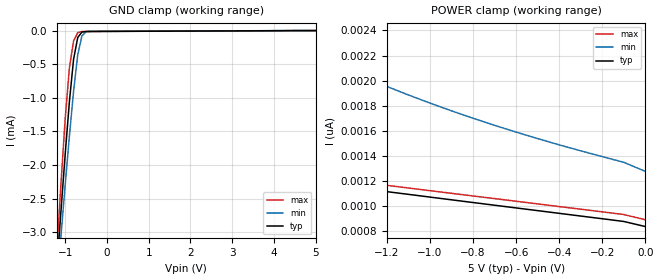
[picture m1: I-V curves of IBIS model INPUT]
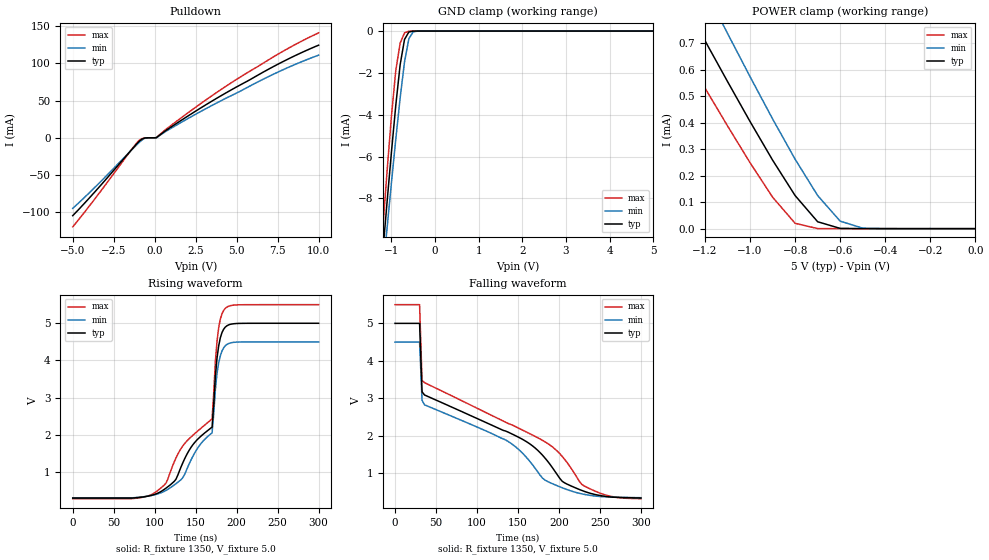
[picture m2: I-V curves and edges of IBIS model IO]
|   PERICOM SEMICONDUCTOR CORP
|   IBIS Model of PI6ULS5V9511A
|   Product Family: ULS
|   MSOP-8 (U) Package
[IBIS Ver] 3.2
[Comment char] |_char
[File Name] pi6uls5v9511a_u_50v.ibs
[File Rev] 1.0
[Source] File originated at Pericom Semiconductor Corp.
[Date] 08/30/2017
[Disclaimer] (C) Copyright PERICOM Semiconductor Corporation
   All rights reserved
  Pericom Semiconductor Corporation hereby grants the user of
  this IBIS model a non-exclusive, nontransferable license to
  use this IBIS model under the following terms.
  This IBIS model is provided on an "AS IS" basis and Pericom
  makes absolutely no warranty with respect to the information
  contained herein. PERICOM DISCLAIMS AND CUSTOMER WAIVES ALL
  WARRANTIES, EXPRESSED OR IMPLIED, INCLUDING WARRANTIES OF
  MERCHANTABILITY OR FITNESS FOR A PARTICULAR PURPOSE. The
  entire risk as to quality and performance is with the customer.
  Accordingly, in no event shall the company be liable for any
  damages, whether in contract or tort, including any lost
  profits or other incidental, consequential, exemplary, or
  punitive damages arising out of the use or application of the
  IBIS model provided in this package. Further, Pericom reserves
  the right to make changes without notice to any product herein
  to improve reliability, function, or design. Pericom does not
  convey any license under patent rights or any other intellectual
  property rights, including those of third parties.
  The user is granted this license only to use the IBIS model
  and is not granted rights to sell, load, rent, lease or license
  the IBIS model in whole or in part, or in modified form to anyone
  other than user. User may modify the IBIS model to suit its specific
  application but rights to derivative works and such modifications
  shall belong to Pericom.
  Pericom is not obligated to provide maintenance or support
  for the licensed IBIS model.
  Contact Pericom at ATTN: APPLICATION ENGINEERING / IBIS MODELS
  1545 Barber Lane Milpitas, CA 95035 USA.
[Component] PI6ULS5V9511A
[Manufacturer] Pericom Semiconductor Corp.
[Package]
| variable   typ   min   max
R_pkg   0.04200   0.03995   0.04405
L_pkg   2.30669n   2.21200n   2.40138n
C_pkg   0.21108p   0.20715p   0.21500p
[Pin] signal_name  model_name   R_pin   L_pin   C_pin
1   ENABLE   INPUT   0.04405   2.40138n   0.21500p
2   SCLOUT   IO   0.03995   2.21200n   0.20715p
3   SCLIN   IO   0.03995   2.21200n   0.20715p
4   GND   GND   0.04405   2.40138n   0.21500p
5   READY   NC   0.04405   2.40138n   0.21500p
6   SDAIN   IO   0.03995   2.21200n   0.20715p
7   SDAOUT   IO   0.03995   2.21200n   0.20715p
8   VCC   POWER   0.04405   2.40138n   0.21500p
| Models and submodels in the file (2): INPUT (Input), IO (Open_drain)
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[Model] INPUT
Model_type Input
Vinl = 1.5000V
Vinh = 3.5000V
| variable   typ   min   max
C_comp   1.600pF   1.560pF   1.640pF
[Voltage Range]   5.0000V   4.5000V   5.5000V
[POWER Clamp Reference] 5.0000V   4.5000V   5.5000V
[GND Clamp Reference]   0.0000V   0.0000V   0.0000V
[Temperature Range]   25   85   -40
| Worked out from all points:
|   GND clamp passes 1 mA (typ) near -0.89 V on its own axis
[GND Clamp]
| Voltage   I(typ)   I(min)   I(max)
-5V       -36.92mA   -32.97mA   -43.67mA
-1.2V     -3.523mA   -3.797mA   -3.27mA
-1.1V     -2.661mA   -3.034mA   -2.251mA
-1V       -1.828mA   -2.287mA   -1.302mA
-900mV    -1.053mA   -1.567mA   -550.5uA
-800mV    -425.6uA   -900.4uA   -153.8uA
-700mV    -102uA     -358.3uA   -30.67uA
-600mV    -22.33uA   -78.81uA   -14.18uA
-500mV    -13.71uA   -18.96uA   -13uA
5V        837.4pA    1.539nA    -201.8pA
[POWER Clamp]
| Voltage   I(typ)   I(min)   I(max)
-5V       2.03nA     9.83nA     1.97nA
-4.4V     1.867nA    7.474nA    1.843nA
-3.5V     1.641nA    4.974nA    1.652nA
-1.8V     1.248nA    2.439nA    1.293nA
-1.7V     1.226nA    2.348nA    1.272nA
-1.4V     1.16nA     2.1nA      1.208nA
-1.2V     1.116nA    1.954nA    1.166nA
-1V       1.073nA    1.821nA    1.124nA
-800mV    1.029nA    1.701nA    1.082nA
-600mV    986.2pA    1.59nA     1.039nA
-100mV    878.2pA    1.349nA    933.7pA
0V        837.7pA    1.277nA    891.7pA
[Model] IO
Model_type Open_drain
Vref=5.000
Rref=1.350E+03
Vmeas=2.50E+00
| variable   typ   min   max
C_comp   4.300E-12   4.290E-12   4.310E-12
[Voltage Range]   5.000E+00   4.500E+00   5.500E+00
[POWER Clamp Reference] 5.000E+00   4.500E+00   5.500E+00
[GND Clamp Reference]   0.000E+00   0.000E+00   0.000E+00
[Pullup Reference]   5.000E+00   4.500E+00   5.500E+00
[Pulldown Reference]   0.000E+00   0.000E+00   0.000E+00
[Temperature Range]   25   85   -40
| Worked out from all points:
|   slope of the pulldown table from 0 to 0.75 V, typ, clamps not added: 69.3 ohm
|   GND clamp passes 1 mA (typ) near -0.75 V on its own axis
|   POWER clamp passes 1 mA (typ) near -1.39 V on its own axis
|   rising waveform, R_fixture 1350, V_fixture 5.0: 20-80 % time 41.9ns typ, 35.5ns min, 50.9ns max; typ from 0.301 V to 5 V
|   falling waveform, R_fixture 1350, V_fixture 5.0: 20-80 % time 156ns typ, 138ns min, 176ns max; typ from 5 V to 0.333 V
[GND Clamp]
| Time   V(typ)   V(min)   V(max)
-5V       -104.6mA   -94.77mA   -119.6mA
-1.2V     -10.63mA   -11.63mA   -9.52mA
-1.1V     -8.183mA   -9.429mA   -6.716mA
-1V       -5.8mA     -7.269mA   -4.08mA
-900mV    -3.55mA    -5.173mA   -1.885mA
-800mV    -1.611mA   -3.196mA   -575.8uA
-700mV    -399.9uA   -1.479mA   -85.6uA
-600mV    -45.37uA   -362.7uA   -5.119uA
-500mV    -3.322uA   -35.76uA   -156.6nA
-400mV    -173.5nA   -2.547uA   -3.218nA
5V        126.9pA    1.739uA    123.8pA
[POWER Clamp]
| Voltage   I(typ)   I(min)   I(max)
-5V       6.861mA    7.517mA    6.252mA
-1.4V     1.023mA    1.241mA    822.9uA
-1.3V     865.9uA    1.071mA    676.4uA
-1.2V     709.9uA    903.6uA    531.2uA
-1.1V     555.7uA    737.5uA    388.2uA
-1V       404.6uA    574uA      249.1uA
-900mV    258.9uA    414.5uA    119uA
-800mV    124.9uA    262.2uA    20.17uA
-700mV    26.02uA    125.1uA    252.6nA
-600mV    923.4nA    28.27uA    1.807nA
-500mV    18.49nA    1.739uA    164.1pA
0V        126.9pA    183.6pA    138.5pA
[Pulldown]
| Voltage   I(typ)   I(min)   I(max)
-5V       -104.6mA   -94.78mA   -119.6mA
-3.5V     -68.93mA   -63.3mA    -77.65mA
-1.4V     -15.73mA   -16.16mA   -15.45mA
-950mV    -4.918mA   -6.353mA   -3.55mA
-800mV    -2.107mA   -3.413mA   -1.333mA
-500mV    -106.5uA   -226.5uA   -70.81uA
100mV     100.4uA    -38.8uA    307.1uA
700mV     10.06mA    8.868mA    11.58mA
2.2V      31.63mA    27.93mA    36.25mA
4.75V     65.28mA    57.45mA    74.97mA
7.6V      99.73mA    89.02mA    113.3mA
10V       124.3mA    111mA      140.9mA
[Rising Waveform]
R_fixture = 1350
V_fixture = 5.0
V_fixture_min = 4.50
V_fixture_max = 5.50
| Time   V(typ)   V(min)   V(max)
0s        301.3mV    309.1mV    286.4mV
84ns      327.7mV    332.5mV    319.4mV
114ns     573.2mV    511.1mV    714.3mV
134ns     1.236V     844.5mV    1.694V
152ns     1.875V     1.633V     2.095V
170ns     2.21V      2.055V     2.432V
174ns     3.568V     3.212V     3.969V
178ns     4.385V     3.931V     4.876V
188ns     4.931V     4.43V      5.434V
300ns     5V         4.5V       5.5V
[Falling Waveform]
R_fixture = 1350
V_fixture = 5.0
V_fixture_min = 4.5
V_fixture_max = 5.5
| Time   V(typ)   V(min)   V(max)
0s        5V         4.501V     5.5V
30ns      5V         4.501V     5.5V
33ns      3.173V     2.946V     3.476V
36ns      3.087V     2.824V     3.417V
138ns     2.094V     1.846V     2.326V
168ns     1.723V     1.216V     2.013V
192ns     1.145V     715.5mV    1.7V
204ns     781mV      607.5mV    1.444V
231ns     510.4mV    430.6mV    653.3mV
300ns     333.1mV    341.5mV    315.3mV
[Ramp]
| variable   typ   min   max
dV/dt_r   2.8195E+00/4.1890E-08  2.5149E+00/3.5519E-08  3.1285E+00/5.0871E-08
dV/dt_f   2.8001E+00/1.5587E-07  2.4925E+00/1.3726E-07  3.1108E+00/1.7551E-07
R_load = 1350
